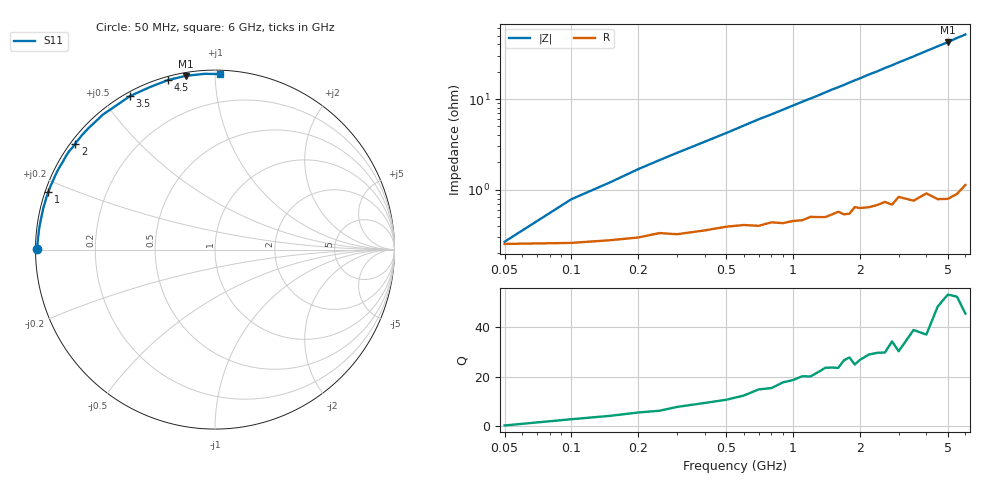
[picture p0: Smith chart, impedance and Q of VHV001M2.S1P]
! Infineon Technologies  Discrete & RF Semiconductors
! BB 814
! Si Tuning Diode in SOT23
! VR =
! S-Parameters:  July  1999
# GHz  S  MA  R  50
!  f  S11
! GHz  MAG  ANG
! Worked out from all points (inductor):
!   34 points, 50 MHz to 6 GHz, reference 50 ohm
!   read as one part to ground: L = 1.32 nH near 150 MHz
!   highest Q = 52.3 at 5 GHz (marker M1), where L = 1.34 nH
!   S11 on the Smith chart (normalised r, x): 50 MHz: 0.01, +0.00; 1 GHz: 0.01, +0.17; 2 GHz: 0.01, +0.34; 3.5 GHz: 0.02, +0.59; 4.5 GHz: 0.02, +0.76; 6 GHz: 0.02, +1.03
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0.05  0.9899 179.8
0.1  0.9897 178.3
0.2  0.9882 176.2
0.3  0.9872 174.2
0.5  0.9846 170.4
0.7  0.9843 166.4
0.8  0.9829 164.6
0.9  0.9834 162.7
1  0.9825 160.8
1.1  0.9823 158.9
1.3  0.9811 155.3
1.5  0.9801 151.5
1.6  0.9789 149.8
1.7  0.9804 148.1
1.8  0.9802 146.2
1.9  0.9769 144.4
2  0.9777 142.8
2.2  0.9777 139.2
2.4  0.9769 136.1
2.6  0.9756 132.6
2.8  0.9778 129.6
3  0.9738 126.3
3.5  0.9778 119.0
4  0.9753 111.9
4.5  0.9803 105.4
5  0.9816 99.6
5.5  0.9811 93.4
6  0.9783 88.4
